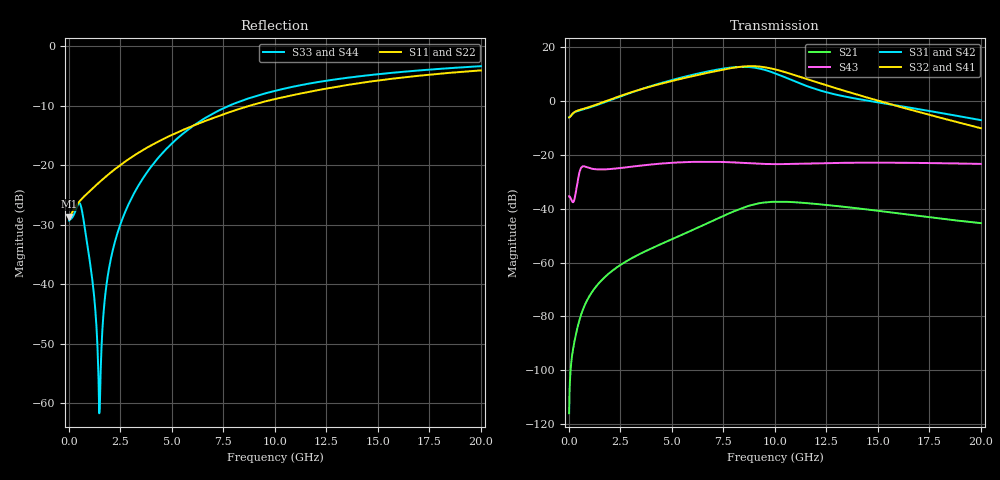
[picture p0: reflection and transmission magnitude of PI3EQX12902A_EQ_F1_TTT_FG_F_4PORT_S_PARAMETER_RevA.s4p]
! NPort=4 DATA=2000 NOISE=0 GROUPDELAY=0 COMPLEX_DATAFORMAT=POLAR
! NumOfBlock=1 NumOfParam=0
! .MODEL Smodel S TSTONEFILE=PI3EQX12902A_EQ_F1_TTT_FG_F_4PORT_S_PARAMETER_RevA.s4p TYPE=S
!  -- The above .MODEL line can be used for the S element in the netlist.
! The s parameter is extracted from the linear redriver, it is not bi-directional; only s(4,1)s(4,2) and s(3,1)s(3,2)
! should be the insertion loss
!Port definition:
!Port1 = input+
!Port2 = input-
!Port3 = output+
!Port4 = output-
# Hz S MA R  50
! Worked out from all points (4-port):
!   2000 points, 10 MHz to 20 GHz, reference 50 ohm
!   strongest paths, dB at 10 MHz, 5.01 GHz, 10.01 GHz, 15.01 GHz, 20 GHz:
!     S32: -6.0, 7.5, 11.8, 0.2, -10.0
!     S41: -6.0, 7.5, 11.7, 0.1, -10.0
!     S31: -6.0, 7.9, 10.3, -0.5, -7.0
!     S42: -6.0, 7.8, 10.2, -0.6, -7.1
!     S43: -35.3, -22.9, -23.4, -22.8, -23.3
!     S21: -116.0, -51.3, -37.3, -40.7, -45.3
!   lowest |S11| = -28.6 dB at 10 MHz (marker M1), VSWR 1.08, Z = 46.4 - j0.0607 ohm
!   |S11| at or under -10 dB: start of sweep to 8.768 GHz
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1e7  0.03704 -179.0  1.589e-06 51.9  0 0.0  0 0.0
     1.589e-06 51.9  0.03704 -179.0  0 0.0  0 0.0
     0.4992 1.1  0.4992 -178.9  0.03429 6.0  0.01709 -177.1
     0.4992 -178.9  0.4992 1.1  0.01709 -177.1  0.03429 6.0
5.78e9  0.2061 -112.0  0.0037 100.2  1.375e-06 -18.3  8.918e-07 90.4
        0.003699 100.2  0.2061 -112.0  8.937e-07 90.6  1.369e-06 -18.1
        2.947 -47.3  2.791 114.0  0.1987 -44.1  0.07366 147.1
        2.781 113.9  2.911 -47.9  0.07404 147.2  0.1981 -44.1
7.68e9  0.2743 -111.6  0.007942 80.6  5.773e-06 -75.0  3.726e-06 46.1
        0.007929 80.5  0.2743 -111.6  3.734e-06 46.1  5.745e-06 -74.6
        4.13 -100.6  3.996 59.7  0.3108 -63.2  0.07326 126.8
        3.972 59.6  4.065 -101.1  0.07373 126.7  0.3101 -63.1
9.11e9  0.3287 -113.2  0.01244 48.5  1.123e-05 -124.1  9.034e-06 -3.9
        0.0124 48.5  0.3287 -113.2  9.026e-06 -4.0  1.118e-05 -123.5
        4.137 -153.6  4.439 5.0  0.3825 -75.1  0.06868 115.4
        4.399 5.0  4.062 -154.0  0.0691 115.2  0.3821 -75.0
1.059e10  0.3788 -115.7  0.01354 11.8  1.475e-05 -164.0  1.428e-05 -61.0
          0.0135 11.9  0.3788 -115.6  1.421e-05 -61.1  1.476e-05 -163.2
          2.679 159.0  3.377 -50.6  0.4454 -84.9  0.0678 108.0
          3.34 -50.3  2.621 158.7  0.06806 107.7  0.4453 -84.8
1.296e10  0.4553 -119.4  0.01132 -26.5  2.208e-05 155.9  1.834e-05 -130.7
          0.01132 -26.2  0.4553 -119.4  1.819e-05 -130.5  2.228e-05 156.6
          1.326 123.8  1.741 -112.1  0.5265 -97.3  0.07127 92.7
          1.726 -111.4  1.293 124.0  0.07124 92.4  0.5269 -97.3
2e10  0.6259 -131.7  0.005375 -75.5  4.067e-05 50.8  1.786e-05 97.5
      0.005425 -75.7  0.6258 -131.7  1.763e-05 98.4  4.115e-05 51.0
      0.4446 37.3  0.3145 131.3  0.6794 -119.6  0.06843 46.2
      0.3158 132.2  0.4392 38.0  0.06833 46.1  0.6797 -119.6
